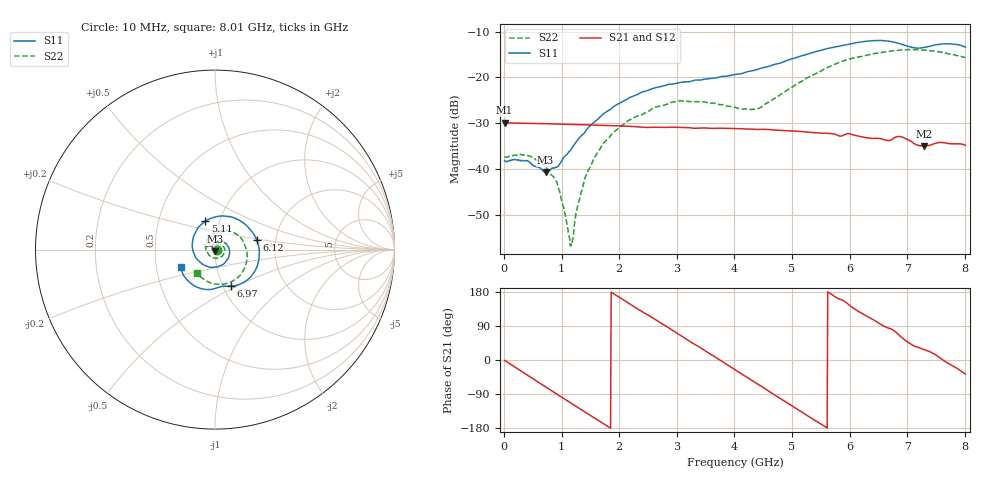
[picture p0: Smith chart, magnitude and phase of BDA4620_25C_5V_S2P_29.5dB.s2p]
!Agilent Technologies,E5071B,MY42404982,A.09.10
!Date: Wed May 06 09:04:53 2026
!Data & Calibration Information:
!Freq	S11:SOLT2(ON)	S21:SOLT2(ON)	S12:SOLT2(ON)	S22:SOLT2(ON)
# Hz S RI R 50
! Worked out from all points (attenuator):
!   801 points, 10 MHz to 8.01 GHz, reference 50 ohm
!   highest |S21| = -29.88 dB at 10 MHz (marker M1); lowest = -34.9 dB at 7.3 GHz (marker M2)
!   lowest |S11| = -40.7 dB at 720 MHz (marker M3), VSWR 1.02, Z = 49.8 - j0.908 ohm
!   |S11| at or under -10 dB: start of sweep to end of sweep
!   |S22| runs from -56.8 to -13.9 dB; largest |S21 - S12| = 0.00017
!   S11 on the Smith chart (normalised r, x): 10 MHz: 1.03, -0.00; 5.11 GHz: 0.86, +0.28; 6.12 GHz: 1.59, +0.18; 6.97 GHz: 1.09, -0.47; 8.01 GHz: 0.67, -0.14
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1e7  0.0124 -0.000799  0.032 -0.000658  0.0321 -0.000673  0.0134 -0.000441
4.4e8  0.00816 -0.00881  0.0229 -0.0217  0.023 -0.0218  0.0131 -0.00479
7.2e8  -0.00156 -0.00911  0.0103 -0.0296  0.0103 -0.0296  0.00833 -0.00679
9.4e8  -0.00984 -0.00437  -0.00117 -0.031  -0.00123 -0.0311  0.00328 -0.00538
1.16e9  -0.0153 0.00585  -0.0123 -0.0282  -0.0123 -0.0283  -0.00124 -0.000761
1.19e9  -0.0157 0.0076  -0.0137 -0.0275  -0.0138 -0.0276  -0.00172 9.8e-05
1.35e9  -0.0159 0.0172  -0.0204 -0.0227  -0.0204 -0.0228  -0.00317 0.00491
1.53e9  -0.0115 0.029  -0.026 -0.0155  -0.0261 -0.0155  -0.00297 0.0114
1.77e9  0.00214 0.0418  -0.0296 -0.00404  -0.0297 -0.00406  0.00117 0.0205
2.15e9  0.0368 0.0459  -0.0257 0.0142  -0.0258 0.0142  0.0173 0.0289
2.68e9  0.0786 0.00544  -0.00578 0.028  -0.00572 0.0281  0.0442 0.019
3.08e9  0.0732 -0.0498  0.0128 0.0255  0.0129 0.0255  0.0549 -0.00748
4.01e9  -0.0713 -0.0803  0.025 -0.012  0.0251 -0.012  -0.0105 -0.0462
4.43e9  -0.1241 -0.00143  0.0111 -0.0248  0.0111 -0.0248  -0.0447 -0.0114
5.11e9  -0.0536 0.1589  -0.0172 -0.0193  -0.0173 -0.0193  -0.0167 0.0853
5.35e9  0.0165 0.1855  -0.0227 -0.0107  -0.0228 -0.0107  0.0232 0.1019
6.12e9  0.2327 0.0536  -0.0153 0.0174  -0.0154 0.0174  0.1612 0.0375
6.68e9  0.1859 -0.1643  0.00218 0.0204  0.00219 0.0205  0.1696 -0.0895
6.97e9  0.0898 -0.2035  0.0135 0.0169  0.0135 0.0169  0.1306 -0.1521
7.3e9  0.0178 -0.2116  0.0159 0.00815  0.016 0.00819  0.0536 -0.191
7.65e9  -0.0987 -0.2103  0.0194 -0.00105  0.0194 -0.00101  -0.0322 -0.1822
8.01e9  -0.1899 -0.0989  0.0146 -0.011  0.0147 -0.011  -0.1025 -0.1282
